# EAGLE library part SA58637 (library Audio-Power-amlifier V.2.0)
The SA58637 is a two-channel audio amplifier in an HVQFN20 package. It provides power output of 2.2 W per channel with an 8 W load at 9 V supply. The internal circuit is comprised of two Bridge-Tied Load (BTL) amplifiers with a complementary PNP-NPN output stage and standby/mute logic. The SA58637 is housed in a 20-pin HVQFN package, which has an exposed die attach paddle enabling reduced thermal resistance and increased power dissipation.
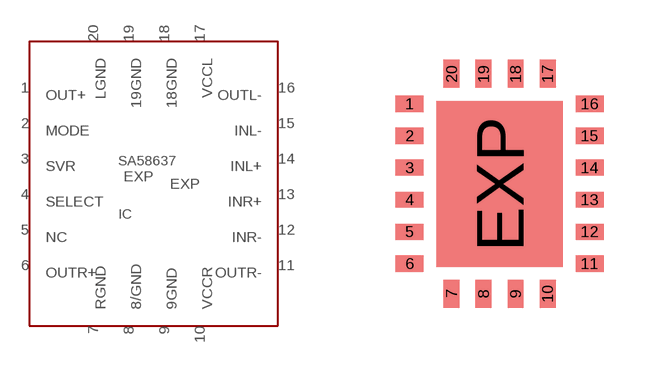
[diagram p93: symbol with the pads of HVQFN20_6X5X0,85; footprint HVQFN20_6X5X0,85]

Designator prefix IC

## SA58637  [HVQFN20_6X5X0,85]
1  OUT+  out
2  MODE
3  SVR
4  SELECT
5  NC  nc
6  OUTR+  out
7  RGND  pwr
8  8/GND  pwr
9  9GND  pwr
10  VCCR  pwr
11  OUTR-  out
12  INR-  in
13  INR+  in
14  INL+  in
15  INL-  in
16  OUTL-  out
17  VCCL  pwr
18  18GND  pwr
19  19GND  pwr
20  LGND  pwr
EXP  EXP  pwr

## Footprint HVQFN20_6X5X0,85 (pad centres in mm)
HVQFN20: plastic thermal enhanced very thin quad flat package; no leads; 20 terminals; body 6 x 5 x 0.85 mm SOT910-1
smd 0.7 x 0.4: 1 -2.25,2; 2 -2.25,1.2; 3 -2.25,0.4; 4 -2.25,-0.4; 5 -2.25,-1.2; 6 -2.25,-2; 11 2.25,-2; 12 2.25,-1.2; 13 2.25,-0.4; 14 2.25,0.4; 15 2.25,1.2; 16 2.25,2
smd 0.4 x 0.7: 7 -1.2,-2.75; 8 -0.4,-2.75; 9 0.4,-2.75; 10 1.2,-2.75; 17 1.2,2.75; 18 0.4,2.75; 19 -0.4,2.75; 20 -1.2,2.75
smd 3.15 x 4.15: EXP 0,-0.01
